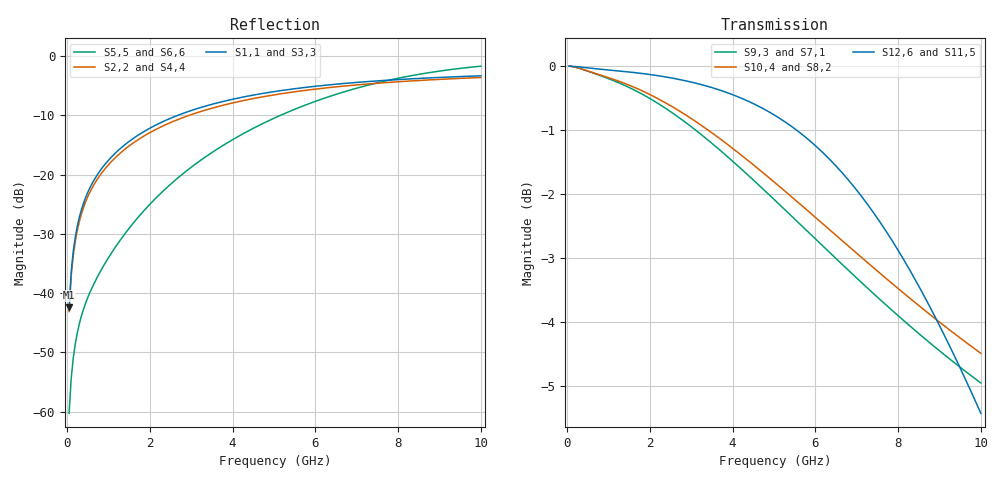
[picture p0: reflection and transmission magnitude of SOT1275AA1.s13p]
! Created Tue Feb  4 22:21:37 2020
! 13 Port Network Data from SP1.SP block
! freq  magS1_1  angS1_1  magS1_2  angS1_2  magS1_3  angS1_3  magS1_4  angS1_4
!  magS1_5  angS1_5  magS1_6  angS1_6  magS1_7  angS1_7  magS1_8  angS1_8
!  magS1_9  angS1_9  magS1_10  angS1_10  magS1_11  angS1_11  magS1_12  angS1_12
!  magS1_13  angS1_13
!  magS2_1  angS2_1  magS2_2  angS2_2  magS2_3  angS2_3
!  magS2_4  angS2_4  magS2_5  angS2_5  magS2_6  angS2_6  magS2_7  angS2_7
!  magS2_8  angS2_8  magS2_9  angS2_9  magS2_10  angS2_10  magS2_11  angS2_11
!  magS2_12  angS2_12  magS2_13  angS2_13
!  magS3_1  angS3_1  magS3_2  angS3_2
!  magS3_3  angS3_3  magS3_4  angS3_4  magS3_5  angS3_5  magS3_6  angS3_6
!  magS3_7  angS3_7  magS3_8  angS3_8  magS3_9  angS3_9  magS3_10  angS3_10
!  magS3_11  angS3_11  magS3_12  angS3_12  magS3_13  angS3_13
!  magS4_1  angS4_1
!  magS4_2  angS4_2  magS4_3  angS4_3  magS4_4  angS4_4  magS4_5  angS4_5
!  magS4_6  angS4_6  magS4_7  angS4_7  magS4_8  angS4_8  magS4_9  angS4_9
!  magS4_10  angS4_10  magS4_11  angS4_11  magS4_12  angS4_12  magS4_13  angS4_13
!  magS5_1  angS5_1  magS5_2  angS5_2  magS5_3  angS5_3  magS5_4  angS5_4
!  magS5_5  angS5_5  magS5_6  angS5_6  magS5_7  angS5_7  magS5_8  angS5_8
!  magS5_9  angS5_9  magS5_10  angS5_10  magS5_11  angS5_11  magS5_12  angS5_12
!  magS5_13  angS5_13
!  magS6_1  angS6_1  magS6_2  angS6_2  magS6_3  angS6_3
!  magS6_4  angS6_4  magS6_5  angS6_5  magS6_6  angS6_6  magS6_7  angS6_7
!  magS6_8  angS6_8  magS6_9  angS6_9  magS6_10  angS6_10  magS6_11  angS6_11
!  magS6_12  angS6_12  magS6_13  angS6_13
!  magS7_1  angS7_1  magS7_2  angS7_2
!  magS7_3  angS7_3  magS7_4  angS7_4  magS7_5  angS7_5  magS7_6  angS7_6
!  magS7_7  angS7_7  magS7_8  angS7_8  magS7_9  angS7_9  magS7_10  angS7_10
!  magS7_11  angS7_11  magS7_12  angS7_12  magS7_13  angS7_13
!  magS8_1  angS8_1
!  magS8_2  angS8_2  magS8_3  angS8_3  magS8_4  angS8_4  magS8_5  angS8_5
!  magS8_6  angS8_6  magS8_7  angS8_7  magS8_8  angS8_8  magS8_9  angS8_9
!  magS8_10  angS8_10  magS8_11  angS8_11  magS8_12  angS8_12  magS8_13  angS8_13
!  magS9_1  angS9_1  magS9_2  angS9_2  magS9_3  angS9_3  magS9_4  angS9_4
!  magS9_5  angS9_5  magS9_6  angS9_6  magS9_7  angS9_7  magS9_8  angS9_8
!  magS9_9  angS9_9  magS9_10  angS9_10  magS9_11  angS9_11  magS9_12  angS9_12
!  magS9_13  angS9_13
!  magS10_1  angS10_1  magS10_2  angS10_2  magS10_3  angS10_3
!  magS10_4  angS10_4  magS10_5  angS10_5  magS10_6  angS10_6  magS10_7  angS10_7
!  magS10_8  angS10_8  magS10_9  angS10_9  magS10_10  angS10_10  magS10_11  angS10_11
!  magS10_12  angS10_12  magS10_13  angS10_13
!  magS11_1  angS11_1  magS11_2  angS11_2
!  magS11_3  angS11_3  magS11_4  angS11_4  magS11_5  angS11_5  magS11_6  angS11_6
!  magS11_7  angS11_7  magS11_8  angS11_8  magS11_9  angS11_9  magS11_10  angS11_10
!  magS11_11  angS11_11  magS11_12  angS11_12  magS11_13  angS11_13
!  magS12_1  angS12_1
!  magS12_2  angS12_2  magS12_3  angS12_3  magS12_4  angS12_4  magS12_5  angS12_5
!  magS12_6  angS12_6  magS12_7  angS12_7  magS12_8  angS12_8  magS12_9  angS12_9
!  magS12_10  angS12_10  magS12_11  angS12_11  magS12_12  angS12_12  magS12_13  angS12_13
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# ghz S ma R 50
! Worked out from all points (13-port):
!   200 points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, 50 MHz to 10 GHz, reference 50 ohm
!   strongest paths, dB at 50 MHz, 2.55 GHz, 5.05 GHz, 7.55 GHz, 10 GHz:
!     S12,6: 0.0, -0.2, -0.8, -2.4, -5.4
!     S11,5: 0.0, -0.2, -0.8, -2.4, -5.4
!     S10,4: 0.0, -0.6, -1.8, -3.2, -4.5
!     S8,2: 0.0, -0.6, -1.8, -3.2, -4.5
!     S9,3: 0.0, -0.7, -2.1, -3.6, -5.0
!     S7,1: 0.0, -0.7, -2.1, -3.6, -5.0
!   lowest |S11| = -42.4 dB at 50 MHz (marker M1), VSWR 1.02, Z = 50 - j0.757 ohm
!   |S11| at or under -10 dB: start of sweep to 2.674 GHz
